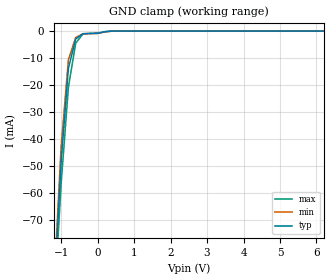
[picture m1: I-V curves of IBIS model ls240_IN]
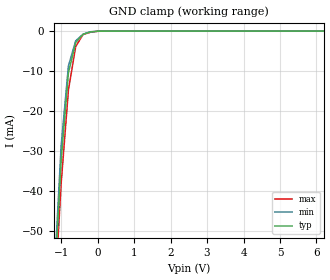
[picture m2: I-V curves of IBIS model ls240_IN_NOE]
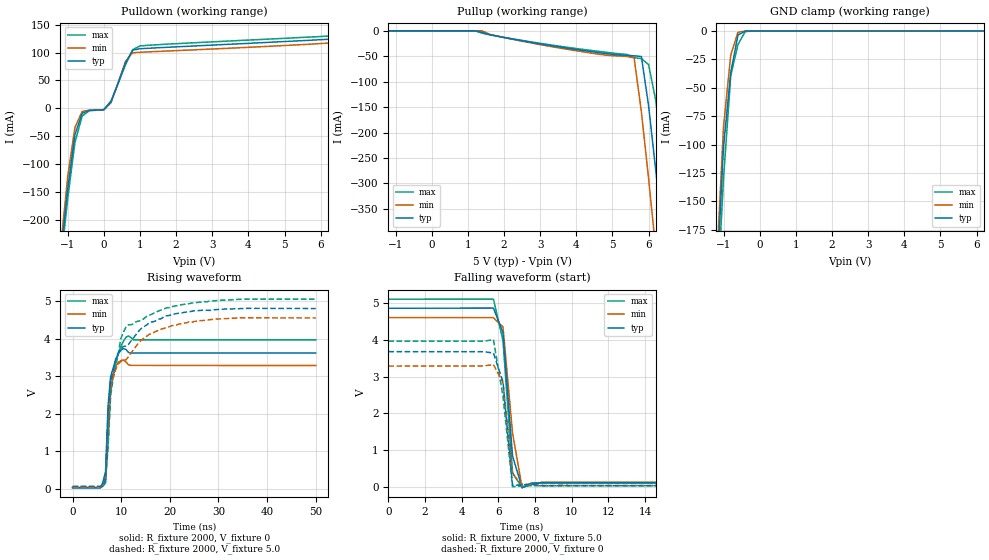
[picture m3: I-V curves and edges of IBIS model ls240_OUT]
|   TEXAS INSTRUMENTS INCORPORATED
|   Standard Linear and Logic Group
|   IBIS Model of SN74LS240
|   OCTAL BUFFERS AND LINE DRIVERS WITH 3-STATE OUTPUTS
|   SOP 20-pin (DW), SOP 20-pin (NS), SSOP 20-pin (DB)
[IBIS Ver]   3.2
[Comment Char]  |_char
[File Name]   sn74ls240.ibs
[File Rev]   3.2
[Date]   November 17, 2004
[Source]   File originated at Texas Instruments, Inc.
[Notes]   The following is a sample IBIS file for the LS240.
   - FILE REV HISTORY
   - 3.2 Re-Release IBIS file on 11/19/04
   - Power clamp data deleted as there is no power-clamp diode
   - All test data contained in this file are derived from
   actual measurements.
   - The measurement used NS package.
   - We have data across voltage and temperature, but not across
   process.
   - File created by Nobuhisa Ohtsubo, SLL Product Engineering.
[Disclaimer] Property of Texas Instruments Incorporated.  Unauthorized
   reproduction and/or distribution is strictly prohibited.
   This product is protected under copyright law.
   Created 2000, (C) Copyright 2000, Texas Instruments Inc.,
   All Rights Reserved.
   UNLESS THERE IS A SIGNED, WRITTEN AGREEMENT TO THE
   CONTRARY, TEXAS INSTRUMENTS () IS PROVIDING THE IBIS
   MODELS  AND WITHOUT ANY WARRANTY, EXPRESSED OR
   IMPLIED.  TI assumes no liability for:
   1) the accuracy of the IBIS models provided to your
   company;
   2) the proper functioning of these IBIS Models in your
   design or for any resulting applications; or
   3) infringement of patents, copyrights or intellectual
   property rights resulting from your use of these IBIS
   models.
   TI provides IBIS Models as a service to our customers.
   You and your company shall not distribute, sell or give
   these models to anyone else without prior written
   permission from TI.
   TI reserves the right to make changes to our products or
   to discontinue any semiconductor product or service
   without notice, and advises our customers to obtain the
   latest version of relevant information to verify, before
   placing orders, that the information being relied on is
   current.
   Please be aware that your receipt and use of the IBIS
   information provided shall serve as acceptance of these
   terms and conditions.  If you do not accept these terms,
   you should return or destroy the IBIS models and any
   other accompanying information immediately.
|   Component ls240_DW
[Component]   ls240_DW
[Manufacturer]  Texas Instruments, Inc.
[Package]
|   typ   min   max
R_pkg   0.038   0.033   0.045
L_pkg   5.012nH   4.110nH   6.349nH
C_pkg   0.717pF   0.530pF   0.868pF
[Pin]   signal_name   model_name   R_pin   L_pin   C_pin
1   1G_NOT   ls240_IN_NOE   0.042   6.336nH   0.865pF
2   1A1   ls240_IN   0.043   5.542nH   0.867pF
3   2Y4   ls240_OUT   0.034   4.714nH   0.732pF
4   1A2   ls240_IN   0.034   4.377nH   0.591pF
5   2Y3   ls240_OUT   0.036   4.130nH   0.533pF
6   1A3   ls240_IN   0.035   4.111nH   0.530pF
7   2Y2   ls240_OUT   0.034   4.284nH   0.583pF
8   1A4   ls240_IN   0.034   4.634nH   0.726pF
9   2Y1   ls240_OUT   0.040   5.518nH   0.865pF
10   GND   GND   0.043   6.349nH   0.866pF
11   2A1   ls240_IN   0.041   6.281nH   0.861pF
12   1Y4   ls240_OUT   0.045   5.561nH   0.868pF
13   2A2   ls240_IN   0.033   4.778nH   0.742pF
14   1Y3   ls240_OUT   0.035   4.414nH   0.596pF
15   2A3   ls240_IN   0.035   4.110nH   0.533pF
16   1Y2   ls240_OUT   0.036   4.130nH   0.533pF
17   2A4   ls240_IN   0.034   4.377nH   0.591pF
18   1Y1   ls240_OUT   0.034   4.714nH   0.731pF
19   2G_NOT   ls240_IN_NOE   0.043   5.569nH   0.868pF
20   VCC   POWER   0.042   6.308nH   0.864pF
|   Component LS240_NS
[Component]   ls240_NS
[Manufacturer]  Texas Instruments, Inc.
[Package]
|   typ   min   max
R_pkg   0.044   0.029   0.058
L_pkg   3.666nH   2.317nH   5.115nH
C_pkg   0.548pF   0.316pF   0.725pF
[Pin]   signal_name   model_name   R_pin   L_pin   C_pin
1   1G_NOT   ls240_IN_NOE   0.058   5.115nH   0.725pF
2   1A1   ls240_IN   0.053   4.591nH   0.724pF
3   2Y4   ls240_OUT   0.049   3.754nH   0.572pF
4   1A2   ls240_IN   0.029   2.549nH   0.388pF
5   2Y3   ls240_OUT   0.031   2.317nH   0.316pF
6   1A3   ls240_IN   0.031   2.317nH   0.316pF
7   2Y2   ls240_OUT   0.029   2.556nH   0.399pF
8   1A4   ls240_IN   0.049   3.754nH   0.579pF
9   2Y1   ls240_OUT   0.053   4.591nH   0.724pF
10   GND   GND   0.058   5.115nH   0.725pF
11   2A1   ls240_IN   0.058   5.115nH   0.725pF
12   1Y4   ls240_OUT   0.053   4.591nH   0.724pF
13   2A2   ls240_IN   0.049   3.754nH   0.579pF
14   1Y3   ls240_OUT   0.029   2.557nH   0.399pF
15   2A3   ls240_IN   0.031   2.317nH   0.316pF
16   1Y2   ls240_OUT   0.031   2.317nH   0.316pF
17   2A4   ls240_IN   0.029   2.557nH   0.399pF
18   1Y1   ls240_OUT   0.049   3.754nH   0.579pF
19   2G_NOT   ls240_IN_NOE   0.053   4.591nH   0.724pF
20   VCC   POWER   0.058   5.115nH   0.725pF
|   Component LS240_DB
[Component]   ls240_DB
[Manufacturer]  Texas Instruments, Inc.
[Package]
|   typ   min   max
R_pkg   0.040   0.035   0.051
L_pkg   3.495nH   3.035nH   4.314nH
C_pkg   0.420pF   0.346pF   0.502pF
[Pin]   signal_name   model_name   R_pin   L_pin   C_pin
1   1G_NOT   ls240_IN_NOE   0.049   4.310nH   0.502pF
2   1A1   ls240_IN   0.048   3.903nH   0.487pF
3   2Y4   ls240_OUT   0.035   3.189nH   0.396pF
4   1A2   ls240_IN   0.035   3.036nH   0.347pF
5   2Y3   ls240_OUT   0.035   3.035nH   0.367pF
6   1A3   ls240_IN   0.035   3.035nH   0.367pF
7   2Y2   ls240_OUT   0.035   3.036nH   0.347pF
8   1A4   ls240_IN   0.035   3.189nH   0.397pF
9   2Y1   ls240_OUT   0.047   3.899nH   0.488pF
10   GND   GND   0.051   4.314nH   0.500pF
11   2A1   ls240_IN   0.051   4.314nH   0.500pF
12   1Y4   ls240_OUT   0.047   3.899nH   0.488pF
13   2A2   ls240_IN   0.035   3.189nH   0.397pF
14   1Y3   ls240_OUT   0.035   3.036nH   0.346pF
15   2A3   ls240_IN   0.035   3.035nH   0.367pF
16   1Y2   ls240_OUT   0.035   3.035nH   0.367pF
17   2A4   ls240_IN   0.035   3.036nH   0.346pF
18   1Y1   ls240_OUT   0.035   3.189nH   0.397pF
19   2G_NOT   ls240_IN_NOE   0.047   3.899nH   0.488pF
20   VCC   POWER   0.051   4.314nH   0.502pF
| Models and submodels in the file (3): ls240_IN (Input), ls240_IN_NOE (Input), ls240_OUT (3-state)
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|   Model ls240_IN
[Model]   ls240_IN
Model_type  Input
Polarity   Inverting
Vinl = 0.8
Vinh = 2.0
| variable   typ   min   max
C_comp   1.33pf   1.00pf   1.66pf
[Temperature Range]   25   0   70
[Voltage Range]   5.0   4.75   5.25
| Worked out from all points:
|   GND clamp passes 1 mA (typ) near -0.40 V on its own axis
[GND Clamp]
|   Voltage   I(typ)   I(min)   I(max)
-5V       -1.265A    -1.347A    -1.142A
-1.2V     -98.98mA   -95.17mA   -103.7mA
-1V       -48.51mA   -42.82mA   -56.74mA
-800mV    -13.8mA    -10.59mA   -20.86mA
-600mV    -2.928mA   -2.339mA   -4.472mA
-400mV    -977.1uA   -976.8uA   -1.043mA
99.48fV   -844.4uA   -859.8uA   -739.2uA
400mV     -1.792uA   -2.176uA   -1.734uA
10V       21.85nA    11.48nA    22.89nA
|   Model ls240_IN_NOE
[Model]   ls240_IN_NOE
Model_type  Input
Polarity   Inverting
Vinl = 0.8
Vinh = 2.0
| variable   typ   min   max
C_comp   1.33pf   1.00pf   1.66pf
[Temperature Range]   25   0   70
[Voltage Range]   5.0   4.75   5.25
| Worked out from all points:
|   GND clamp passes 1 mA (typ) near -0.42 V on its own axis
[GND Clamp]
|   Voltage   I(typ)   I(min)   I(max)
-5V       -891.1mA   -939.4mA   -814.1mA
-1.2V     -66.35mA   -63.23mA   -70.31mA
-1V       -32.39mA   -28.67mA   -38.19mA
-800mV    -10.45mA   -8.682mA   -14.75mA
-600mV    -2.866mA   -2.422mA   -3.861mA
-400mV    -795.8uA   -789uA     -872.4uA
-200mV    -224.1uA   -174uA     -300.5uA
200mV     -24.02uA   -24.66uA   -22.27uA
10V       21.55nA    7.48nA     16.74nA
|   Model ls240_OUT
[Model]   ls240_OUT
Model_type  3-state
Polarity   Non-Inverting
Enable   Active-Low
Vmeas = 1.3v
Cref = 45pf
Rref = 667
Vref = 0V
| variable   typ   min   max
C_comp   5.8pf   4.35pf   7.25pf
[Temperature Range]   25   0   70
[Voltage Range]   5.0   4.75   5.25
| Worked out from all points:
|   slope of the pulldown table from 0 to 0.75 V, typ, clamps not added: 7.43 ohm
|   GND clamp passes 1 mA (typ) near -0.46 V on its own axis
|   rising waveform, R_fixture 2000, V_fixture 0: 20-80 % time 895ps typ, 799ps min, 1.53ns max; typ from 0.032 V to 3.62 V
|   falling waveform, R_fixture 2000, V_fixture 5.0: 20-80 % time 442ps typ, 561ps min, 476ps max; typ from 4.86 V to 0.116 V
|   rising waveform, R_fixture 2000, V_fixture 5.0: 20-80 % time 4.53ns typ, 5.18ns min, 2.82ns max; typ from 0.07 V to 4.8 V
|   falling waveform, R_fixture 2000, V_fixture 0: 20-80 % time 448ps typ, 408ps min, 590ps max; typ from 3.68 V to 0.034 V
[Pulldown]
|   Voltage   I(typ)   I(min)   I(max)
-5V       -2.684A    -2.902A    -2.499A
-1.2V     -269.1mA   -253mA     -282.7mA
-1V       -144.1mA   -122.3mA   -162mA
-800mV    -47.38mA   -34.28mA   -61.3mA
-600mV    -8.857mA   -5.476mA   -13.73mA
-400mV    -3.498mA   -3.302mA   -4.04mA
0V        -2.461mA   -2.752mA   -2.219mA
200mV     12.21mA    10.01mA    13.37mA
600mV     81.14mA    84.41mA    78.46mA
800mV     104.3mA    99.62mA    105.1mA
1V        106.8mA    100.4mA    111.8mA
10V       140mA      132.2mA    144.2mA
[Pullup]
|   Voltage   I(typ)   I(min)   I(max)
-5V       2.341uA    270.6nA    6.315uA
1.2V      -2.603uA   88.24nA    -103.2uA
1.4V      -3.155mA   -83.56uA   -4.822mA
3.2V      -28.02mA   -29.66mA   -26.78mA
5.4V      -48.03mA   -50.37mA   -46.46mA
5.6V      -49.11mA   -53.46mA   -52.89mA
5.8V      -50.43mA   -159.1mA   -54.6mA
6V        -147.5mA   -290.7mA   -66.46mA
6.2V      -276mA     -431.8mA   -137.5mA
6.4V      -403.7mA   -572.8mA   -253.7mA
6.6V      -534.5mA   -710.2mA   -377.9mA
10V       -2.607A    -3A        -2.31A
[GND Clamp]
|   Voltage   I(typ)   I(min)   I(max)
-5V       -3.151A    -3.374A    -2.719A
-1.2V     -228.5mA   -212.3mA   -250.6mA
-1V       -101.9mA   -84.41mA   -130mA
-800mV    -36.46mA   -21.12mA   -39.14mA
-600mV    -3.452mA   -1.046mA   -11.86mA
-400mV    -16.16uA   -2.085uA   -445.9uA
-200mV    -166.6nA   -17.58nA   -2.72uA
10V       215uA      239.2uA    176.9uA
[Ramp]
| variable   typ   min   max
dV/dt_r  2.088E+00/3.133E-09  1.878E+00/2.562E-09  2.322E+00/5.549E-09
dV/dt_f  2.964E+00/1.635E-09  2.808E+00/1.908E-09  3.132E+00/1.564E-09
[Rising Waveform]
R_fixture = 2000
V_fixture = 0
V_fixture_min = 0
V_fixture_max = 0
C_fixture = 0pf
L_fixture = 0nH
|   Time   V(typ)   V(min)   V(max)
0s        31.83mV    43.21mV    29.46mV
5.729ns   31.86mV    43.37mV    29.49mV
6.771ns   452.4mV    305.1mV    160.9mV
7.292ns   2.217V     1.849V     1.228V
7.813ns   2.989V     2.853V     2.581V
9.375ns   3.595V     3.371V     3.6V
10.42ns   3.735V     3.434V     3.925V
11.46ns   3.636V     3.306V     4.073V
12.5ns    3.62V      3.287V     3.965V
50ns      3.618V     3.285V     3.965V
[Falling Waveform]
R_fixture = 2000
V_fixture = 5.0
V_fixture_min = 4.75
V_fixture_max = 5.25
C_fixture = 0pf
L_fixture = 0nH
|   Time   V(typ)   V(min)   V(max)
0s        4.862V     4.608V     5.108V
5.729ns   4.866V     4.605V     5.11V
6.25ns    4.198V     4.351V     3.98V
6.771ns   840.5mV    1.466V     388.6mV
7.292ns   -16.91mV   -17.67mV   -24.25mV
7.813ns   78.97mV    65.84mV    111.3mV
8.333ns   116.5mV    129mV      107.3mV
50ns      115.9mV    129.2mV    108mV
[Rising Waveform]
R_fixture = 2000
V_fixture = 5.0
V_fixture_min = 4.75
V_fixture_max = 5.25
C_fixture = 0pf
L_fixture = 0nH
|   Time   V(typ)   V(min)   V(max)
0s        70mV       47.6mV     61.01mV
5.729ns   70.05mV    52.5mV     61.89mV
6.771ns   252.1mV    257.8mV    238.3mV
7.292ns   2.005V     1.645V     1.119V
7.813ns   2.859V     2.675V     2.471V
9.896ns   3.72V      3.389V     3.994V
11.46ns   3.843V     3.509V     4.367V
15.63ns   4.403V     4.105V     4.617V
23.96ns   4.713V     4.446V     4.93V
50ns      4.801V     4.551V     5.051V
[Falling Waveform]
R_fixture = 2000
V_fixture = 0
V_fixture_min = 0
V_fixture_max = 0
C_fixture = 0pf
L_fixture = 0nH
|   Time   V(typ)   V(min)   V(max)
0s        3.681V     3.288V     3.967V
5.208ns   3.68V      3.293V     3.966V
5.729ns   3.643V     3.329V     4.008V
6.25ns    2.861V     2.834V     2.465V
6.771ns   41.58mV    347.4mV    6.79mV
7.292ns   58.98mV    75.46mV    26.84mV
7.813ns   69.63mV    71.67mV    35.42mV
8.333ns   32.92mV    45.74mV    31.01mV
50ns      33.75mV    44.02mV    33.62mV
